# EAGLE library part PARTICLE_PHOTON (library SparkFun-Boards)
Particle Photon Footprint of the Particle Photon that is used as a basis for many Photon shields. SparkFun Products: Particle Photon SparkFun Photon ProtoShield SparkFun Photon micro OLED Shield SparkFun Photon IMU Shield SparkFun Photon Battery Shield
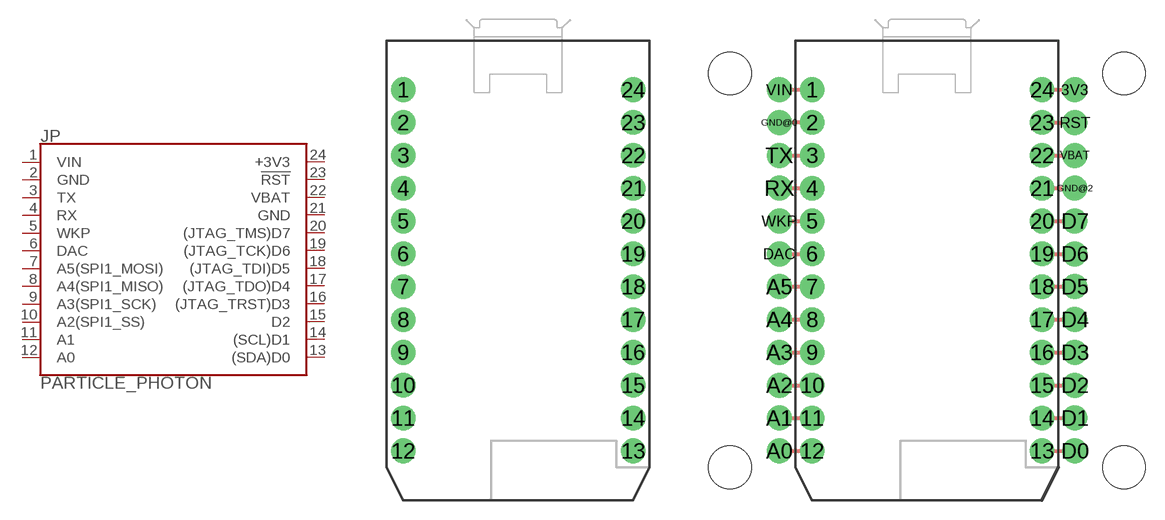
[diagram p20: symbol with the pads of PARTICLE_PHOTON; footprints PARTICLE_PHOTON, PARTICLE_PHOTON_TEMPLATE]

Designator prefix JP

## PARTICLE_PHOTON  [PARTICLE_PHOTON]
1  VIN  pwr
2  GND  pwr
3  TX
4  RX
5  WKP
6  DAC
7  A5(SPI1_MOSI)
8  A4(SPI1_MISO)
9  A3(SPI1_SCK)
10  A2(SPI1_SS)
11  A1
12  A0
13  (SDA)D0
14  (SCL)D1
15  D2
16  (JTAG_TRST)D3
17  (JTAG_TDO)D4
18  (JTAG_TDI)D5
19  (JTAG_TCK)D6
20  (JTAG_TMS)D7
21  GND  pwr
22  VBAT  pwr
23  !RST!
24  +3V3  pwr

## PARTICLE_PHOTONTEMPLATE  [PARTICLE_PHOTON_TEMPLATE]
1  VIN  pwr
2  GND  pwr
3  TX
3V3  +3V3  pwr
4  RX
5  WKP
6  DAC
7  A5(SPI1_MOSI)
8  A4(SPI1_MISO)
9  A3(SPI1_SCK)
10  A2(SPI1_SS)
11  A1
12  A0
13  (SDA)D0
14  (SCL)D1
15  D2
16  (JTAG_TRST)D3
17  (JTAG_TDO)D4
18  (JTAG_TDI)D5
19  (JTAG_TCK)D6
20  (JTAG_TMS)D7
21  GND  pwr
22  VBAT  pwr
23  !RST!
24  +3V3  pwr
A0  A0
A1  A1
A2  A2(SPI1_SS)
A3  A3(SPI1_SCK)
A4  A4(SPI1_MISO)
A5  A5(SPI1_MOSI)
D0  (SDA)D0
D1  (SCL)D1
D2  D2
D3  (JTAG_TRST)D3
D4  (JTAG_TDO)D4
D5  (JTAG_TDI)D5
D6  (JTAG_TCK)D6
D7  (JTAG_TMS)D7
DAC  DAC
GND@0  GND  pwr
GND@2  GND  pwr
RST  !RST!
RX  RX
TX  TX
VBAT  VBAT  pwr
VIN  VIN  pwr
WKP  WKP

## PARTICLE_PHOTONTEMPLATE_WIDE  [PARTICLE_PHOTON_TEMPLATE_WIDE]
Pads as for PARTICLE_PHOTON_TEMPLATE

## PARTICLE_PHOTONTEMPLATE_NO_STANDOFF  [PARTICLE_PHOTON_TEMPLATE_NO_STANDOFF]
Pads as for PARTICLE_PHOTON_TEMPLATE

## Footprint PARTICLE_PHOTON (pad centres in mm)
Particle Photon Specifications: Pin count: 24 Pin pitch:0.1" Area: 0.8 x 1.4 inches Example device(s): Particle Photon
drill 1.016 pad 1.905: 1 -8.89,13.97; 2 -8.89,11.43; 3 -8.89,8.89; 4 -8.89,6.35; 5 -8.89,3.81; 6 -8.89,1.27; 7 -8.89,-1.27; 8 -8.89,-3.81; 9 -8.89,-6.35; 10 -8.89,-8.89; 11 -8.89,-11.43; 12 -8.89,-13.97; 13 8.89,-13.97; 14 8.89,-11.43; 15 8.89,-8.89; 16 8.89,-6.35; 17 8.89,-3.81; 18 8.89,-1.27; 19 8.89,1.27; 20 8.89,3.81; 21 8.89,6.35; 22 8.89,8.89; 23 8.89,11.43; 24 8.89,13.97

## Footprint PARTICLE_PHOTON_TEMPLATE (pad centres in mm)
Particle Photon Template Used for laying out a shield that breaks out Photon pins. Specifications: Pin count:48 Pin pitch:0.1" Area: 0.8 x 1.4 inches Example device(s): Particle Photon
drill 1.016 pad 1.905: 1 -8.89,13.97; 2 -8.89,11.43; 3 -8.89,8.89; 4 -8.89,6.35; 5 -8.89,3.81; 6 -8.89,1.27; 7 -8.89,-1.27; 8 -8.89,-3.81; 9 -8.89,-6.35; 10 -8.89,-8.89; 11 -8.89,-11.43; 12 -8.89,-13.97; 13 8.89,-13.97; 14 8.89,-11.43; 15 8.89,-8.89; 16 8.89,-6.35; 17 8.89,-3.81; 18 8.89,-1.27; 19 8.89,1.27; 20 8.89,3.81; 21 8.89,6.35; 22 8.89,8.89; 23 8.89,11.43; 24 8.89,13.97
drill 1.016 pad 1.93: 3V3 11.43,13.97; A0 -11.43,-13.97; A1 -11.43,-11.43; A2 -11.43,-8.89; A3 -11.43,-6.35; A4 -11.43,-3.81; A5 -11.43,-1.27; D0 11.43,-13.97; D1 11.43,-11.43; D2 11.43,-8.89; D3 11.43,-6.35; D4 11.43,-3.81; D5 11.43,-1.27; D6 11.43,1.27; D7 11.43,3.81; DAC -11.43,1.27; GND@0 -11.43,11.43; GND@2 11.43,6.35; RST 11.43,11.43; RX -11.43,6.35; TX -11.43,8.89; VBAT 11.43,8.89; VIN -11.43,13.97; WKP -11.43,3.81
hole 3.302 at -15.24,15.24
hole 3.302 at 15.24,15.24
hole 3.302 at -15.24,-15.24
hole 3.302 at 15.24,-15.24

## Footprint PARTICLE_PHOTON_TEMPLATE_WIDE (pad centres in mm)
Particle Photon Template wIDE Used for laying out a shield that breaks out Photon pins with 0.2" spacing. Specifications: Pin count:48 Pin pitch:0.1" Area: 1.6 x 1.4 inches Example device(s):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
drill 1.016 pad 1.905: 1 -8.89,13.97; 2 -8.89,11.43; 3 -8.89,8.89; 4 -8.89,6.35; 5 -8.89,3.81; 6 -8.89,1.27; 7 -8.89,-1.27; 8 -8.89,-3.81; 9 -8.89,-6.35; 10 -8.89,-8.89; 11 -8.89,-11.43; 12 -8.89,-13.97; 13 8.89,-13.97; 14 8.89,-11.43; 15 8.89,-8.89; 16 8.89,-6.35; 17 8.89,-3.81; 18 8.89,-1.27; 19 8.89,1.27; 20 8.89,3.81; 21 8.89,6.35; 22 8.89,8.89; 23 8.89,11.43; 24 8.89,13.97
drill 1.016 pad 1.93: 3V3 13.97,13.97; A0 -13.97,-13.97; A1 -13.97,-11.43; A2 -13.97,-8.89; A3 -13.97,-6.35; A4 -13.97,-3.81; A5 -13.97,-1.27; D0 13.97,-13.97; D1 13.97,-11.43; D2 13.97,-8.89; D3 13.97,-6.35; D4 13.97,-3.81; D5 13.97,-1.27; D6 13.97,1.27; D7 13.97,3.81; DAC -13.97,1.27; GND@0 -13.97,11.43; GND@2 13.97,6.35; RST 13.97,11.43; RX -13.97,6.35; TX -13.97,8.89; VBAT 13.97,8.89; VIN -13.97,13.97; WKP -13.97,3.81
hole 3.302 at -17.78,15.24
hole 3.302 at 17.78,15.24
hole 3.302 at -17.78,-15.24
hole 3.302 at 17.78,-15.24

## Footprint PARTICLE_PHOTON_TEMPLATE_NO_STANDOFF (pad centres in mm)
drill 1.016 pad 1.905: 1 -8.89,12.7; 2 -8.89,10.16; 3 -8.89,7.62; 4 -8.89,5.08; 5 -8.89,2.54; 6 -8.89,0; 7 -8.89,-2.54; 8 -8.89,-5.08; 9 -8.89,-7.62; 10 -8.89,-10.16; 11 -8.89,-12.7; 12 -8.89,-15.24; 13 8.89,-15.24; 14 8.89,-12.7; 15 8.89,-10.16; 16 8.89,-7.62; 17 8.89,-5.08; 18 8.89,-2.54; 19 8.89,0; 20 8.89,2.54; 21 8.89,5.08; 22 8.89,7.62; 23 8.89,10.16; 24 8.89,12.7
drill 1.016 pad 1.93: 3V3 11.43,12.7; A0 -11.43,-15.24; A1 -11.43,-12.7; A2 -11.43,-10.16; A3 -11.43,-7.62; A4 -11.43,-5.08; A5 -11.43,-2.54; D0 11.43,-15.24; D1 11.43,-12.7; D2 11.43,-10.16; D3 11.43,-7.62; D4 11.43,-5.08; D5 11.43,-2.54; D6 11.43,0; D7 11.43,2.54; DAC -11.43,0; GND@0 -11.43,10.16; GND@2 11.43,5.08; RST 11.43,10.16; RX -11.43,5.08; TX -11.43,7.62; VBAT 11.43,7.62; VIN -11.43,12.7; WKP -11.43,2.54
